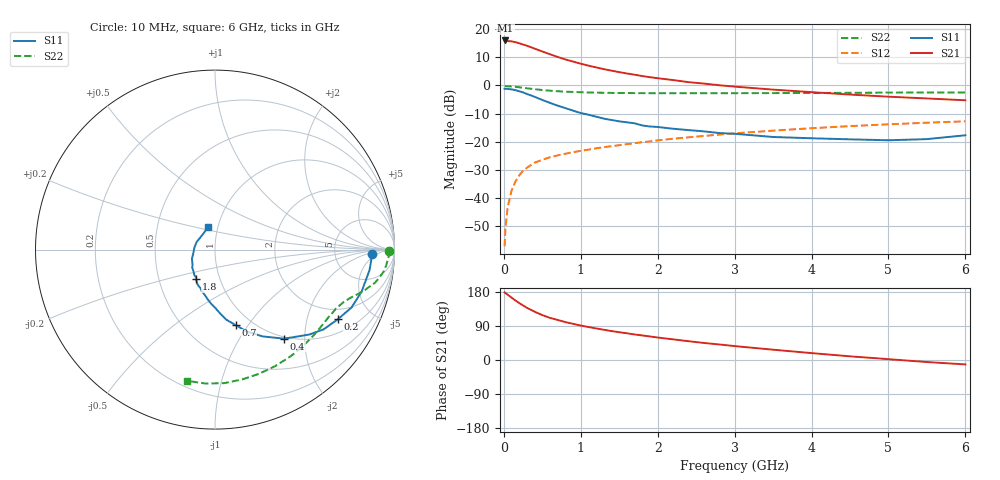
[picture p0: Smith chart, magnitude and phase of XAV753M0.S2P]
! SIEMENS Discrete & RF Semiconductors
! BFY180
! Si NPN RF Bipolar Junction Transistor in MICRO-X
! VCE = 0.75 V  IC = 3 mA
! Common Emitter S-Parameters:  May  1997
# GHz  S  MA  R  50
!  f  S11  S21  S12  S22
! GHz  MAG  ANG  MAG  ANG  MAG  ANG  MAG  ANG
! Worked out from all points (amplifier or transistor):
!   36 points, 10 MHz to 6 GHz, reference 50 ohm
!   highest |S21| = 16.0 dB at 20 MHz (marker M1)
!   |S21| within 3 dB of that: start of sweep to 409.4 MHz
!   unconditionally stable (mu >= 1): 679.3 MHz to end of sweep
!   at 250 MHz: K = 0.43, MSG = 22.4 dB, |S12| = -30.3 dB
!   at 1.4 GHz: K = 1.51, MAG = 9.2 dB, |S12| = -21.6 dB
!   at 6 GHz: K = 1.69, MAG = -1.1 dB, |S12| = -12.7 dB
!   S11 on the Smith chart (normalised r, x): 10 MHz: 14, -3; 200 MHz: 1.52, -3.11; 400 MHz: 0.97, -1.59; 700 MHz: 0.84, -0.88; 1.8 GHz: 0.77, -0.26; 6 GHz: 0.89, +0.22
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0.01  0.8724 -1.6  6.178 178.6  0.0014 90.6  0.9689 -0.5
0.02  0.8737 -3.1  6.286 176.7  0.0028 87.9  0.9739 -1.1
0.05  0.8684 -7.6  6.135 172.4  0.0069 81.8  0.9671 -2.6
0.1  0.8499 -15.9  6.061 164.6  0.0135 80.9  0.958 -5.3
0.15  0.8262 -23.0  5.859 157.2  0.0196 75.7  0.9457 -7.7
0.2  0.7872 -29.5  5.604 150.2  0.0253 71.4  0.9274 -9.8
0.3  0.7062 -42.1  5.068 137.7  0.0345 64.5  0.8896 -13.2
0.4  0.628 -52.2  4.499 127.5  0.0425 59.6  0.8573 -15.7
0.5  0.552 -61.2  4.008 118.5  0.0478 56.0  0.8288 -17.6
0.6  0.4901 -68.7  3.575 111.1  0.0531 53.8  0.8062 -19.2
0.7  0.4369 -74.6  3.205 105.7  0.0573 52.0  0.7889 -20.7
0.8  0.3959 -80.8  2.891 100.0  0.0612 51.2  0.7752 -22.0
0.9  0.3571 -85.4  2.652 95.5  0.0653 50.0  0.7655 -23.4
1.1  0.302 -94.2  2.243 87.1  0.0724 49.3  0.7497 -26.0
1.4  0.2434 -107.7  1.828 76.3  0.0832 48.1  0.7364 -30.5
1.8  0.1948 -122.5  1.466 64.8  0.0984 46.8  0.73 -36.5
2.2  0.1702 -134.9  1.245 54.5  0.113 44.6  0.7278 -42.8
2.8  0.1428 -152.7  1.008 41.0  0.1341 41.1  0.7278 -52.1
3.5  0.1215 -171.6  0.843 27.2  0.1575 36.1  0.7307 -62.8
4.5  0.1104 157.1  0.688 9.7  0.1894 28.0  0.739 -78.2
5.5  0.1114 123.8  0.587 -5.4  0.2179 19.6  0.7481 -94.0
6  0.1303 108.4  0.545 -11.6  0.2306 15.1  0.7475 -102.0
